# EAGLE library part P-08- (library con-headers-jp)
HEADER PLUG PINS
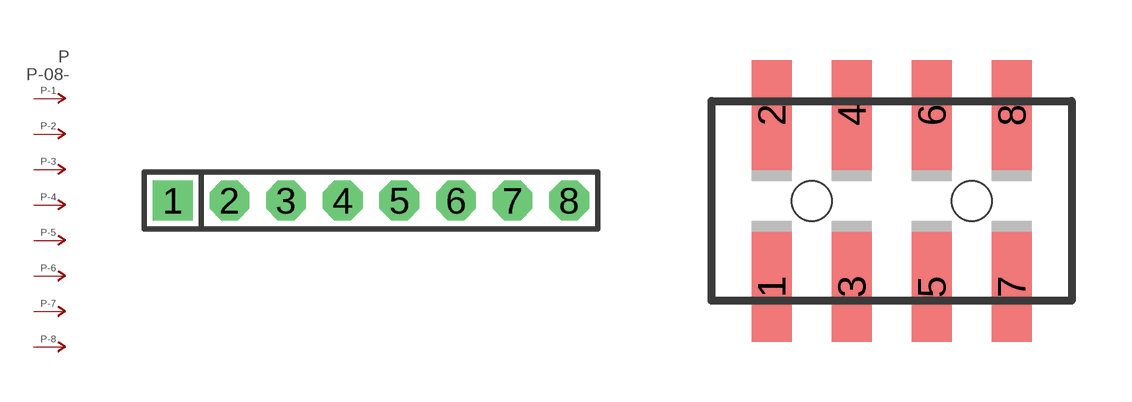
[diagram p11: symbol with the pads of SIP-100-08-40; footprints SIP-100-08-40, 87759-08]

Designator prefix P; gates -2=P-N -3=P-N -4=P-N -5=P-N -6=P-N -7=P-N -8=P-N -1=P-NV

## P-08-SIP-100-40  [SIP-100-08-40]
1  -1:P  pas
2  -2:P  pas
3  -3:P  pas
4  -4:P  pas
5  -5:P  pas
6  -6:P  pas
7  -7:P  pas
8  -8:P  pas

## P-08-87759  [87759-08]
Pads as for SIP-100-08-40

## P-08-100-2X04  [DIL-100-2X04]
Pads as for SIP-100-08-40

## P-08-2MM-2X04  [DIL-2MM-2X04]
Pads as for SIP-100-08-40

## P-08-100-2X04_M  [DIL-100-2X04_M]
Pads as for SIP-100-08-40

## P-08-2MM-2X04_M  [DIL-2MM-2X04_M]
Pads as for SIP-100-08-40

## P-08-SIP-100-32  [SIP-100-08-32]
Pads as for SIP-100-08-40

## P-08-SIP-100-40Y  [SIP-100-08-40Y]
Pads as for SIP-100-08-40

## P-08-SIP-100-32Y  [SIP-100-08-32Y]
Pads as for SIP-100-08-40

## P-08-87759_M  [87759-08_M]
Pads as for SIP-100-08-40

## P-08-LCW-108-XX-X-S  [LCW-108-XX-X-S]
Pads as for SIP-100-08-40

## P-08-LCW-108-XX-X-S-RE  [LCW-108-XX-X-S-RE]
Pads as for SIP-100-08-40

## Footprint SIP-100-08-40 (pad centres in mm)
SIP Header - 0.1", 40 mil drill
drill 1.016 pad 1.778 square: 1 -8.89,0
drill 1.016 pad 1.778 octagon: 2 -6.35,0; 3 -3.81,0; 4 -1.27,0; 5 1.27,0; 6 3.81,0; 7 6.35,0; 8 8.89,0

## Footprint 87759-08 (pad centres in mm)
Molex PCB Pin Headers 2.00mm (.079") Pitch Milli-Grid Header, Vertical SMD
smd 1 x 2.75: 1 -3,-2.15; 2 -3,2.15; 3 -1,-2.15; 4 -1,2.15; 5 1,-2.15; 6 1,2.15; 7 3,-2.15; 8 3,2.15
hole 1 at -2,0
hole 1 at 2,0

## Footprint DIL-100-2X04 (pad centres in mm)
PIN HEADER - 0.1"
drill 1.016 square: 1 -3.81,-1.27
drill 1.016 octagon: 2 -3.81,1.27; 3 -1.27,-1.27; 4 -1.27,1.27; 5 1.27,-1.27; 6 1.27,1.27; 7 3.81,-1.27; 8 3.81,1.27

## Footprint DIL-2MM-2X04 (pad centres in mm)
PIN HEADER - 2MM"
drill 0.711 square: 1 -3,-1
drill 0.711: 2 -3,1; 3 -1,-1; 4 -1,1; 5 1,-1; 6 1,1; 7 3,-1; 8 3,1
